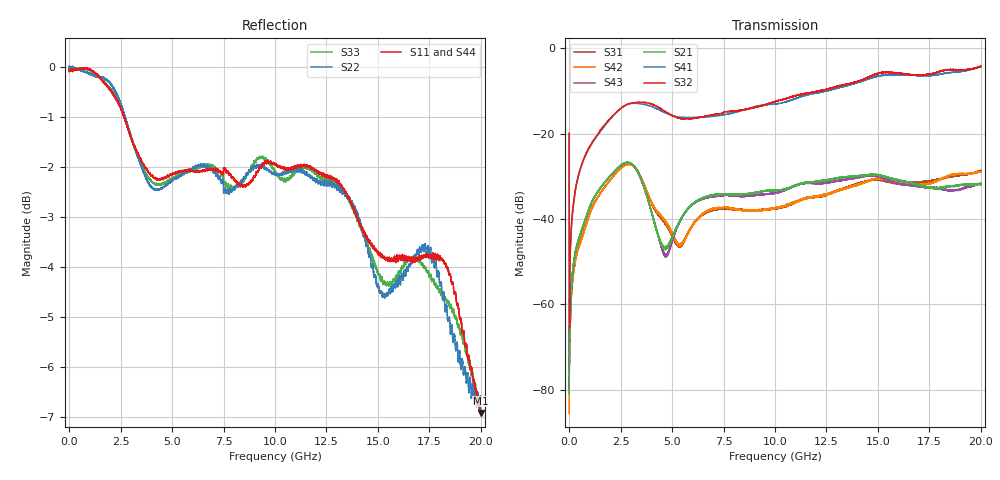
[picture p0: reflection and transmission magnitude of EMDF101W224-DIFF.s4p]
!EMDF101W224
!Johanson Technology Inc.
!www.johansontechnology.com
!Test Board Conditions:
!Substrate Type  RO4350B
!Substrate Thickness  21 mil
!Substrate Dk  3.66
!TL Type: GCPW
!TL Trace Width  40 mil
!TL Gap  17.5 mil
!PART MODE DIFFERENTIAL
!DUT TOPOLOGY	DIFFERENTIAL 4-PORT
# MHz S  dB  R 50
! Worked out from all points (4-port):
!   20001 points, 300 kHz to 20 GHz, reference 50 ohm
!   strongest paths, dB at 300 kHz, 5 GHz, 10 GHz, 15 GHz, 20 GHz:
!     S32: -19.9, -15.8, -12.5, -6.0, -4.2
!     S41: -19.9, -15.8, -13.1, -6.6, -4.4
!     S21: -81.1, -44.3, -33.3, -29.7, -32.0
!     S43: -65.0, -45.2, -33.8, -30.0, -31.7
!     S42: -85.6, -43.4, -37.5, -30.6, -29.0
!     S31: -72.7, -44.0, -37.6, -30.8, -28.7
!   lowest |S11| = -6.9 dB at 20 GHz (marker M1), VSWR 2.64, Z = 30.3 - j34 ohm
!   |S11| at or under -10 dB: nowhere
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0.3  -0.09 -174.2  -73.50 -49.4  -67.29 -19.1  -19.89 -83.5
     -81.05 -79.9  -0.02 -174.3  -19.98 -83.6  -71.43 -48.2
     -72.70 -68.9  -19.93 -83.5  -0.09 -174.3  -75.04 -46.9
     -19.95 -83.5  -85.57 -27.7  -65.05 -24.2  0.03 -174.2
440.293  -0.04 173.5  -45.25 75.0  -46.93 71.7  -30.09 76.4
         -45.21 74.3  -0.04 173.3  -30.00 77.2  -47.08 70.7
         -47.07 70.8  -30.00 76.8  -0.03 173.2  -45.13 72.3
         -30.13 76.6  -46.97 71.5  -45.16 73.1  0.00 172.4
2687.26  -1.02 136.3  -26.91 -7.5  -27.29 -15.0  -13.49 23.2
         -26.90 -7.3  -0.95 138.4  -13.54 25.4  -27.52 -13.7
         -27.29 -15.2  -13.52 25.1  -1.01 136.4  -26.93 -9.6
         -13.49 23.3  -27.52 -13.7  -26.96 -9.3  -1.01 136.2
4689.23  -2.21 122.4  -46.89 -35.3  -41.32 -96.5  -15.21 -33.1
         -46.85 -34.3  -2.37 118.5  -14.89 -35.0  -40.64 -96.0
         -41.10 -95.8  -14.88 -35.2  -2.31 119.3  -48.87 -42.7
         -15.20 -32.6  -40.77 -95.1  -48.67 -41.2  -2.25 117.8
11930.12  -2.06 25.7  -31.34 -92.0  -34.88 -128.7  -10.60 -83.2
          -31.30 -92.5  -2.23 28.3  -10.18 -82.2  -34.84 -126.2
          -34.85 -129.6  -10.26 -81.3  -2.12 20.6  -31.75 -99.7
          -10.57 -84.1  -34.79 -126.6  -31.61 -100.6  -2.20 20.7
19997  -6.92 -97.1  -32.26 73.9  -28.60 44.3  -4.54 146.8
       -31.92 74.8  -6.61 -96.7  -3.97 148.8  -28.89 47.1
       -28.67 45.1  -4.20 149.3  -6.91 -106.2  -31.96 64.2
       -4.34 146.2  -28.96 45.8  -31.81 61.9  -6.79 -103.4
20000  -6.92 -97.2  -32.20 73.9  -28.66 44.5  -4.52 146.7
       -31.98 74.5  -6.62 -96.6  -4.01 148.8  -28.95 47.1
       -28.68 44.7  -4.21 149.2  -6.92 -106.2  -31.96 63.4
       -4.35 146.2  -28.98 45.9  -31.73 61.7  -6.78 -103.4
